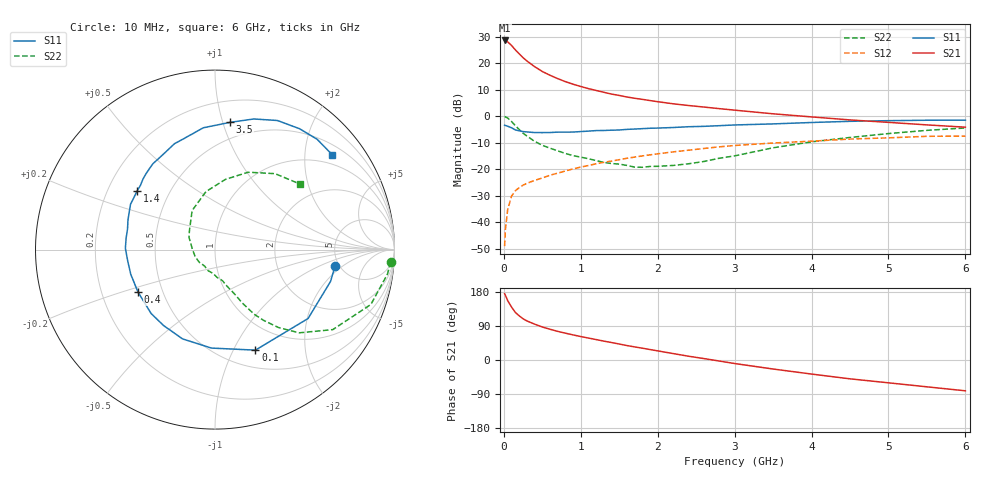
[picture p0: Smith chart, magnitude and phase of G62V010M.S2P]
! SIEMENS Small Signal Semiconductors
! BFG193
! Si NPN RF Bipolar Junction Transistor in SOT223
! VCE = 2 V  IC = 10 mA
! Common Emitter S-Parameters:  August  1996
# GHz  S  MA  R  50
!  f  S11  S21  S12  S22
! GHz  MAG  ANG  MAG  ANG  MAG  ANG  MAG  ANG
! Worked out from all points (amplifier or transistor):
!   36 points, 10 MHz to 6 GHz, reference 50 ohm
!   highest |S21| = 28.6 dB at 10 MHz (marker M1)
!   |S21| within 3 dB of that: start of sweep to 133.3 MHz
!   unconditionally stable (mu >= 1): 846.7 MHz to 2.691 GHz
!   at 250 MHz: K = 0.54, MSG = 24.1 dB, |S12| = -26.1 dB
!   at 1.4 GHz: K = 1.07, MAG = 11.0 dB, |S12| = -17.0 dB
!   at 6 GHz: K = 0.91, MSG = 1.7 dB, |S12| = -7.5 dB
!   S11 on the Smith chart (normalised r, x): 10 MHz: 4.63, -1.54; 100 MHz: 0.70, -1.23; 400 MHz: 0.36, -0.22; 1.4 GHz: 0.33, +0.30; 3.5 GHz: 0.37, +1.06; 6 GHz: 0.74, +2.64
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0.01  0.6754 -7.7  26.92 175.0  0.0035 96.1  0.9816 -4.0
0.02  0.6678 -15.4  26.7 171.0  0.0072 83.9  0.9704 -8.1
0.05  0.6452 -36.5  25.29 156.7  0.0172 73.4  0.9207 -19.4
0.1  0.6037 -68.1  21.68 139.8  0.0309 62.7  0.7932 -34.2
0.15  0.549 -92.1  17.86 125.4  0.039 54.4  0.6592 -44.7
0.2  0.5293 -110.0  15.02 116.5  0.0447 51.5  0.5605 -50.8
0.25  0.5109 -124.1  12.73 108.8  0.0497 49.2  0.477 -55.6
0.3  0.5035 -135.0  11.03 103.1  0.0539 48.3  0.4207 -58.8
0.4  0.4899 -151.3  8.607 94.6  0.0611 48.4  0.3346 -62.9
0.5  0.4891 -163.8  6.983 87.1  0.068 48.1  0.2814 -65.5
0.6  0.4906 -173.0  5.922 81.1  0.0766 49.0  0.2484 -68.0
0.7  0.4993 179.2  5.121 75.6  0.0838 49.0  0.2213 -71.0
0.9  0.5009 166.6  4.014 66.2  0.1008 48.3  0.1798 -76.1
1.1  0.5214 156.5  3.312 57.9  0.1169 47.2  0.1571 -85.0
1.4  0.5431 143.2  2.613 46.1  0.1419 43.7  0.1275 -100.7
1.7  0.571 132.4  2.178 34.6  0.1686 39.5  0.1091 -120.8
2.2  0.6102 116.5  1.713 17.0  0.2114 30.1  0.1172 -162.0
2.8  0.661 100.0  1.387 -2.7  0.2632 18.0  0.1603 154.8
3.5  0.7141 83.2  1.108 -23.8  0.3109 1.6  0.2525 120.3
4.5  0.7989 64.2  0.849 -49.7  0.3693 -18.0  0.3958 81.5
5.5  0.8375 47.2  0.684 -70.8  0.4163 -41.6  0.5393 51.7
6  0.8402 39.0  0.619 -81.3  0.421 -55.1  0.5982 37.6
